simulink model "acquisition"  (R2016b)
settings: Solver=ode45  StartTime=0.0  StopTime=35*3600  RelTol=1e-3  EnableMultiTasking=on
undefined symbols (not defined in the file or in its folder): drhe, drhi, dte, dti, dto, serial
libraries: instrumentlib x3

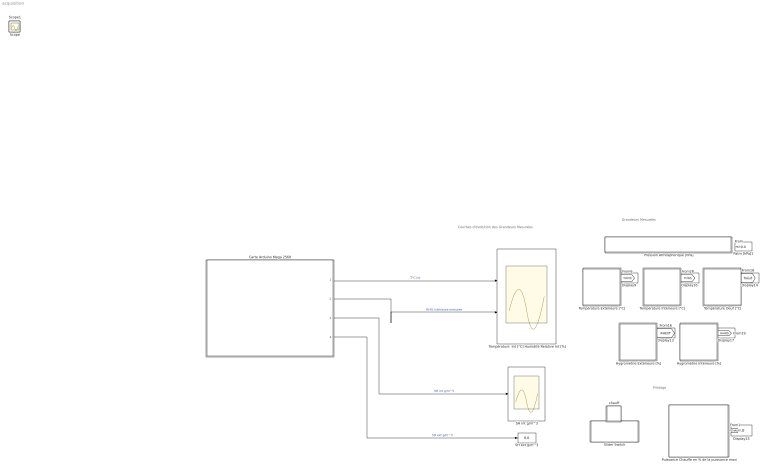
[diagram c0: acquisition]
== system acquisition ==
  note: Grandeurs Mesurées
  note: Pilotage
  note: Courbes d'évolution des Grandeurs Mesurées
  Carte Arduino Mega 2560 : Subsystem
  Display{9,13..17} (6 alike) : Display
  Hygrométrie Extérieure [%] : Subsystem  DialogController=hmiCreateDDGDialog  IsWebBlock=on
  Hygrométrie Intérieure [%] : Subsystem  DialogController=hmiCreateDDGDialog  IsWebBlock=on
  Patm [hPa]1 : Display
  Pression Atmosphérique [hPa] : Subsystem  DialogController=hmiCreateDDGDialog  IsWebBlock=on
  Puissance Chauffe en % de la puissance maxi : Subsystem  DialogController=hmiCreateDDGDialog  IsWebBlock=on
  SH ext g/m^3 : Display
  SH int g/m^3 : Scope
  Slider Switch : Subsystem  DialogController=hmiCreateDDGDialog  IsWebBlock=on
  Température Extérieure [°C] : Subsystem  DialogController=hmiCreateDDGDialog  IsWebBlock=on
  Température Intérieure [°C] : Subsystem  DialogController=hmiCreateDDGDialog  IsWebBlock=on
  Température  Int [°C] Humidité Relative Int [%] : Scope  NumInputPorts=2
  Température Oeuf [°C] : Subsystem  DialogController=hmiCreateDDGDialog  IsWebBlock=on
  chauff : Subsystem  DialogController=hmiCreateDDGDialog  IsWebBlock=on
  Scope : Scope
  Scope1 : Scope
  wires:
  Carte Arduino Mega 2560/1(T°C int) -> Température  Int [°C] Humidité Relative Int [%]/1  "T°C int"
  Carte Arduino Mega 2560/2(RHint) -> Température  Int [°C] Humidité Relative Int [%]/2  "RH% intérieure mesurée"
  [PCHAUFF] -> Display15/1
  [TCINT] -> Display16/1
  [PATM] -> Patm [hPa]1/1
  [TCEXT] -> Display9/1
  [Toeuf] -> Display14/1
  [RHINT] -> Display17/1
  [RHEXT] -> Display13/1
  Carte Arduino Mega 2560/4(SH EXT) -> SH ext g/m^3/1  "SH ext g/m^3"
  Carte Arduino Mega 2560/3(SH INT) -> SH int g/m^3/1  "SH int g/m^3"

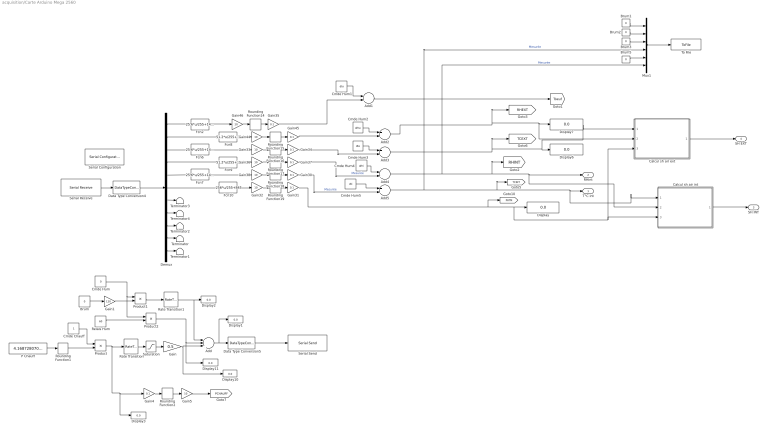
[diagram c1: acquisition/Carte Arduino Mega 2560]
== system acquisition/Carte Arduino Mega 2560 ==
  Add : Sum  Inputs=+++
  Add{1..5} (5 alike) : Sum
  Brum{,1..3,5} (5 alike) : Constant  Value=0  SampleTime=1
  Calcul sh air ext : MATLAB Function  TreatAsAtomicUnit=on
  Calcul sh air int : MATLAB Function  TreatAsAtomicUnit=on
  Cmde Chauff : Constant  SampleTime=1
  Cmde Hum : Constant  Value=0  SampleTime=1
  Cmde Hum1 : Constant  Value=dto  SampleTime=1
  Cmde Hum2 : Constant  Value=drhe  SampleTime=1
  Cmde Hum3 : Constant  Value=dte  SampleTime=1
  Cmde Hum4 : Constant  Value=drhi  SampleTime=1
  Cmde Hum5 : Constant  Value=dti  SampleTime=1
  Data Type Conversion4 : DataTypeConversion  OutDataTypeStr=double
  Data Type Conversion5 : DataTypeConversion  OutDataTypeStr=uint8
  Demux : Demux  Outputs=11
  Display{,1..3,6..7,10..11} (8 alike) : Display
  Fcn10 : Fcn  Expr=256*u/255+845
  Fcn2 : Fcn  Expr=25.6*u/255+14.4
  Fcn6 : Fcn  Expr=25.6*u/255+14.4
  Fcn7 : Fcn  Expr=25.6*u/255+14.4
  Fcn8 : Fcn  Expr=51.2*u/255+35
  Fcn9 : Fcn  Expr=51.2*u/255+35
  Gain : Gain  Gain=0.5
  Gain1 : Gain  Gain=120
  Gain{4,30..31,34..35,37,45} (7 alike) : Gain  Gain=0.1
  Gain{5,32..33,36,38,44,46} (7 alike) : Gain  Gain=10
  Mux1 : Mux  Inputs=6
  P Chauff : Constant  Value=4.1687280703799  SampleTime=1
  Product : Product
  Product1 : Product
  Product2 : Product
  Rate Transition : RateTransition  OutPortSampleTime=1
  Rate Transition1 : RateTransition  OutPortSampleTime=1
  Relais Hum : Constant  Value=60  SampleTime=1
  Rounding Function{1..2,14..19} (8 alike) : Rounding  Operator=round
  Saturation : Saturate  UpperLimit=100  LowerLimit=1
  Serial Configuration : instrumentlib/Serial Configuration  Priority=-200000  ComPortMenu=<Please select a port...>  ComPort=COM8  ObjConstructor=serial('COM8');  BaudRate=9600  DataBits=8  Parity=none  StopBits=1  FlowControl=none  Timeout=10  ByteOrder=LittleEndian
  Serial Receive : instrumentlib/Serial Receive  ComPortMenu=<Please select a port...>  ComPort=COM8  ObjConstructor=serial('COM8');  Terminator=<none>  DataSize="[1  11]"  DataType=uint8  EnableBlockingMode=on  ActionDataUnavailable=Output last received value  CustomValue=0  SampleTime=1
  Serial Send : instrumentlib/Serial Send  ComPortMenu=<Please select a port...>  ComPort=COM8  ObjConstructor=serial('COM8');  Terminator=<none>  EnableBlockingMode=on
  Terminator{,1..4} (5 alike) : Terminator
  To File : ToFile  Filename=acqui.mat  SaveFormat=Timeseries
  T°C int : Outport
  RHint : Outport  Port=2
  SH INT : Outport  Port=3
  SH EXT : Outport  Port=4
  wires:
  Mux1/1 -> To File/1
  Gain35/1 -> Add1/2
  Add2/1 -> Calcul sh air ext/2(rh), Display7/1, [RHEXT]
  Add4/1 -> Mux1/6, RHint/1, Calcul sh air int/2(rh), [RHINT]  "Mesurée"
  Add3/1 -> Calcul sh air ext/1(T), Display6/1, [TCEXT]
  Demux/2 -> Fcn8/1
  Demux/3 -> Fcn6/1
  Demux/4 -> Fcn9/1
  Demux/5 -> Fcn7/1
  Demux/1 -> Fcn2/1
  Fcn2/1 -> Gain46/1
  Fcn6/1 -> Gain33/1
  Fcn7/1 -> Gain38/1
  Fcn8/1 -> Gain44/1
  Fcn9/1 -> Gain36/1
  Fcn10/1 -> Gain32/1
  Rounding Function14/1 -> Gain35/1
  Gain46/1 -> Rounding Function14/1
  Rounding Function15/1 -> Gain45/1
  Gain44/1 -> Rounding Function15/1
  Rounding Function16/1 -> Gain34/1
  Gain33/1 -> Rounding Function16/1
  Rounding Function17/1 -> Gain37/1
  Gain36/1 -> Rounding Function17/1
  Rounding Function18/1 -> Gain30/1
  Gain38/1 -> Rounding Function18/1
  Rounding Function19/1 -> Gain31/1
  Gain32/1 -> Rounding Function19/1
  Serial Receive/1 -> Data Type Conversion4/1
  Data Type Conversion4/1 -> Demux/1
  Demux/6 -> Fcn10/1
  Add5/1 -> Mux1/4, Calcul sh air int/1(T), T°C int/1, [TCINT]  "Mesurée"
  Gain/1 -> Display10/1, Add/3
  Demux/10 -> Terminator/1
  Demux/11 -> Terminator1/1
  Demux/9 -> Terminator2/1
  Data Type Conversion5/1 -> Serial Send/1
  Rate Transition/1 -> Saturation/1
  Cmde Chauff/1 -> Product/1
  Product/1 -> Display3/1, Gain4/1, Rate Transition/1
  Add/1 -> Display1/1, Data Type Conversion5/1
  Cmde Hum/1 -> Product2/1, Product1/1
  Brum/1 -> Gain1/1
  Gain1/1 -> Product1/2
  Product1/1 -> Rate Transition1/1
  Rate Transition1/1 -> Display2/1, Add/1
  Relais Hum/1 -> Product2/2
  Product2/1 -> Display11/1, Add/2
  Gain31/1 -> [PATM], Calcul sh air ext/3(pl), Calcul sh air int/3(pl), Display/1
  Demux/7 -> Terminator3/1
  Demux/8 -> Terminator4/1
  Brum1/1 -> Mux1/1
  Brum2/1 -> Mux1/2
  Brum3/1 -> Mux1/3
  Brum5/1 -> Mux1/5
  Calcul sh air ext/1(sh) -> SH EXT/1
  Calcul sh air int/1(sh) -> SH INT/1
  Rounding Function1/1 -> Product/2
  P Chauff/1 -> Rounding Function1/1
  Gain4/1 -> Rounding Function2/1
  Rounding Function2/1 -> Gain5/1
  Gain5/1 -> [PCHAUFF]
  Add1/1 -> [Toeuf]
  Cmde Hum1/1 -> Add1/1
  Gain45/1 -> Add2/2
  Cmde Hum2/1 -> Add2/1
  Cmde Hum3/1 -> Add3/1
  Gain34/1 -> Add3/2
  Cmde Hum4/1 -> Add4/1
  Gain37/1 -> Add4/2  "Mesurée"
  Gain30/1 -> Add5/2  "Mesurée"
  Cmde Hum5/1 -> Add5/1
  Saturation/1 -> Gain/1

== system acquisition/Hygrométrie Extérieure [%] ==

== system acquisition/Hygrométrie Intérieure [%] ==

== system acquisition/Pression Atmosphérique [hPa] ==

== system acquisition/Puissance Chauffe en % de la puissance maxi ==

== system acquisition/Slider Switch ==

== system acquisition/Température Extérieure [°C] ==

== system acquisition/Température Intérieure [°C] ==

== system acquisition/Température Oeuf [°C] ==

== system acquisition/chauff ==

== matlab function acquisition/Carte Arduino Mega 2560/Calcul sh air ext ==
function sh =CONV_RH_en_SH(T,rh,pl)

% ######################################################################################################
% function [sh]=goff_gratch(T,rh,pl)
%
% fonction de conversion de l'humidité relative ('rh' : en %)
% en humidité spécifique ('sh' : en g/m^3)
% en fonction de :
% la temperature de l'air ('T' : Kelvin, utiliser la fonction C2K si la T est en °C)
% du niveau pression ('pl' : en hPa, si vous avez des matrices 4D, bouclez sur la dimension 
% niveau). 
%
% utilise l'equation de Goff-Gratch pour la determination de
% la tension de vapeur saturante (es) en fonction de la temperature de l'Air
%
% AUTHOR : Nicolas Fauchereau - CRC Dijon - <nicolasf@u-bourgogne.fr>
%
% ######################################################################################################



%Conversion température
T=T+273.2;


% tension de vapeur saturante
if (T<0), % par rapport a la glace 
eilog = -9.09718 .* ((273.16 ./ T) -1);
eilog2 = -3.5654 .* log10 (273.16 ./ T);
eilog3 = 0.876793 .* (1 - (T ./ 273.16 ));
es=6.1071 .* 10.^(eilog+eilog2+eilog3);

else, % par rapport à l'eau 
eilog=-7.90298 .* ((373.16 ./ T) - 1);
eilog2=5.02808 .* log10((373.16 ./ T));
eilog3=-1.3816e-7 .* ((10.^(11.344.*(1-(T./373.16)))) -1);
eilog4=8.1328e-3 .* ((10.^( -3.49149 .* ((373.16 ./ T) - 1) )) -1);
es=1013.246 .* 10.^(eilog+eilog2+eilog3+eilog4);
end;


% masse
ws = 0.62197 .* es ./ (pl - 0.378.*es);

% masse volumique
ro = 1.293 .* 273 ./ (T);

% humidité spécifique
sh = (rh/100.0)*ws;
sh=sh*1000*ro; %%% passage en g.m^3

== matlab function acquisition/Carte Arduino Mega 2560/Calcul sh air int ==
function sh =CONV_RH_en_SH(T,rh,pl)

% ######################################################################################################
% function [sh]=goff_gratch(T,rh,pl)
%
% fonction de conversion de l'humidité relative ('rh' : en %)
% en humidité spécifique ('sh' : en g/m^3)
% en fonction de :
% la temperature de l'air ('T' : Kelvin, utiliser la fonction C2K si la T est en °C)
% du niveau pression ('pl' : en hPa, si vous avez des matrices 4D, bouclez sur la dimension 
% niveau). 
%
% utilise l'equation de Goff-Gratch pour la determination de
% la tension de vapeur saturante (es) en fonction de la temperature de l'Air
%
% AUTHOR : Nicolas Fauchereau - CRC Dijon - <nicolasf@u-bourgogne.fr>
%
% ######################################################################################################



%Conversion température
T=T+273.2;


% tension de vapeur saturante
if (T<0), % par rapport a la glace 
eilog = -9.09718 .* ((273.16 ./ T) -1);
eilog2 = -3.5654 .* log10 (273.16 ./ T);
eilog3 = 0.876793 .* (1 - (T ./ 273.16 ));
es=6.1071 .* 10.^(eilog+eilog2+eilog3);

else, % par rapport à l'eau 
eilog=-7.90298 .* ((373.16 ./ T) - 1);
eilog2=5.02808 .* log10((373.16 ./ T));
eilog3=-1.3816e-7 .* ((10.^(11.344.*(1-(T./373.16)))) -1);
eilog4=8.1328e-3 .* ((10.^( -3.49149 .* ((373.16 ./ T) - 1) )) -1);
es=1013.246 .* 10.^(eilog+eilog2+eilog3+eilog4);
end;


% masse
ws = 0.62197 .* es ./ (pl - 0.378.*es);

% masse volumique
ro = 1.293 .* 273 ./ (T);

% humidité spécifique
sh = (rh/100.0)*ws;
sh=sh*1000*ro; %%% passage en g.m^3
